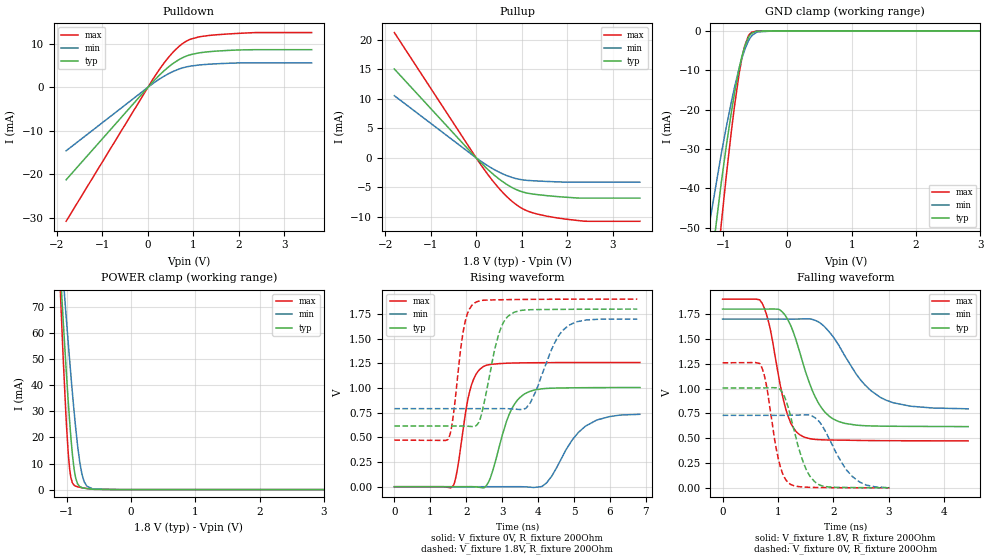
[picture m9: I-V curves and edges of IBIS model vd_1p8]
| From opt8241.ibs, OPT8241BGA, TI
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|   vd_1p8 Model
[Model]   vd_1p8
Model_type   I/O
Polarity   Non-Inverting
Enable   Active-Low
Vinl = 0.54
Vinh = 1.26
Vmeas = 0.9
Vref = 0
Cref = 2pF
Rref = 300
|   typ   min   max
|   (nom PVT)   (fast PVT)   (slow PVT)
C_comp   2.314e-12   2.106e-12   2.515e-12
[Model spec]
|subparameter
Vinl   0.54   0.51   0.57
Vinh   1.26   1.19   1.33
| Where nom  PVT is Nominal Process, 1.8V, 27C
|   Fast PVT is Strong Process,  1.9V, -40C
|   Slow PVT is Weak Process,   1.7V, 125C
[Voltage Range]   1.8   1.7   1.9
|Junction Temperature
[Temperature Range]   27   125   -40
[Pullup Reference]   1.8   1.7   1.9
[Pulldown Reference]   0   0   0
[Power Clamp Reference]   1.8   1.7   1.9
[GND Clamp Reference]   0   0   0
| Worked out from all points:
|   slope of the pulldown table from 0 to 0.27 V, typ, clamps not added: 90.7 ohm
|   slope of the pullup table from 0 to 0.27 V, typ, clamps not added: 131 ohm
|   GND clamp passes 1 mA (typ) near -0.58 V on its own axis
|   POWER clamp passes 1 mA (typ) near -0.78 V on its own axis
|   falling waveform, V_fixture 1.8V, R_fixture 200Ohm: 20-80 % time 451ps typ, 685ps min, 306ps max; typ from 1.8 V to 0.617 V
|   rising waveform, V_fixture 0V, R_fixture 200Ohm: 20-80 % time 523ps typ, 792ps min, 341ps max; typ from 0 V to 1 V
|   rising waveform, V_fixture 1.8V, R_fixture 200Ohm: 20-80 % time 422ps typ, 606ps min, 286ps max; typ from 0.614 V to 1.8 V
|   falling waveform, V_fixture 0V, R_fixture 200Ohm: 20-80 % time 309ps typ, 448ps min, 225ps max; typ from 1.01 V to 0.002 V
[Pulldown]
|   Voltage   I(typ)   I(min)   I(max)
-1.8V     -21.3mA    -14.64mA   -30.86mA
138.6mV   1.594mA    1.077mA    2.336mA
321.6mV   3.491mA    2.343mA    5.13mA
467.8mV   4.81mA     3.206mA    7.084mA
579.6mV   5.682mA    3.765mA    8.38mA
736.5mV   6.676mA    4.382mA    9.863mA
943.6mV   7.528mA    4.886mA    11.09mA
1.147V    7.957mA    5.151mA    11.65mA
1.464V    8.296mA    5.386mA    12.05mA
2.379V    8.654mA    5.601mA    12.6mA
3.6V      8.654mA    5.601mA    12.6mA
[GND Clamp]
|   Voltage   I(typ)   I(min)   I(max)
-1.8V     -229.4mA   -136.4mA   -324.1mA
-1.234V   -65.48mA   -50.91mA   -83.76mA
-1.03V    -38.61mA   -31.28mA   -49.11mA
-872.8mV  -20.69mA   -18.03mA   -25.55mA
-756.2mV  -9.942mA   -9.797mA   -11.38mA
-710.3mV  -6.6mA     -7.091mA   -7.076mA
-663.8mV  -3.897mA   -4.757mA   -3.745mA
-604.9mV  -1.604mA   -2.501mA   -1.231mA
-552.6mV  -571.6uA   -1.205mA   -335.5uA
-474mV    -83.6uA    -300.2uA   -29.97uA
-180mV    0A         -257.9nA   0A
3.6V      0A         0A         0A
[Pullup]
|   Voltage   I(typ)   I(min)   I(max)
-1.8V     15.04mA    10.52mA    21.2mA
127.8mV   -1.011mA   -694.5uA   -1.444mA
340.3mV   -2.541mA   -1.729mA   -3.653mA
510.4mV   -3.613mA   -2.435mA   -5.227mA
682.2mV   -4.533mA   -3.019mA   -6.61mA
863.8mV   -5.298mA   -3.474mA   -7.809mA
1.049V    -5.821mA   -3.744mA   -8.708mA
1.246V    -6.112mA   -3.865mA   -9.296mA
1.563V    -6.39mA    -3.983mA   -9.866mA
1.976V    -6.655mA   -4.105mA   -10.36mA
2.389V    -6.795mA   -4.106mA   -10.71mA
3.6V      -6.795mA   -4.106mA   -10.72mA
[POWER Clamp]
|   Voltage   I(typ)   I(min)   I(max)
-1.8V     411mA      341.7mA    540.9mA
-1.105V   86.59mA    98.07mA    80.06mA
-1.067V   70.27mA    85.51mA    57.79mA
-1.012V   47.3mA     67.39mA    28.39mA
-975.5mV  33.65mA    56.1mA     13.87mA
-935.5mV  20.27mA    44.06mA    4.743mA
-880.3mV  7.155mA    28.72mA    1.602mA
-831mV    2.23mA     16.99mA    1.098mA
-763mV    752.5uA    5.919mA    741.6uA
-688.2mV  401uA      1.367mA    429.5uA
-599.2mV  175.8uA    309.4uA    159uA
3.6V      0A         0A         0A
[Ramp]
R_load = 200
|   typ   min   max
dV/dt_r   0.603657/5.22202e-10   0.438286/7.7537e-10   0.755458/3.39341e-10
dV/dt_f   0.711295/4.52207e-10   0.545564/6.91155e-10   0.856494/3.0524e-10
[Falling Waveform]
V_fixture = 1.8V
V_fixture_min = 1.7V
V_fixture_max = 1.9V
R_fixture = 200Ohm
|   Time   V(typ)   V(min)   V(max)
0s        1.8V       1.7V       1.9V
712ps     1.8V       1.7V       1.86V
858ps     1.8V       1.7V       1.605V
1.152ns   1.718V     1.7V       771.6mV
1.396ns   1.359V     1.7V       533.7mV
1.722ns   861.5mV    1.674V     486.3mV
2.092ns   668.7mV    1.44V      481.3mV
2.51ns    627.9mV    1.074V     477.6mV
2.95ns    621.2mV    883mV      475.5mV
4.43ns    617.3mV    796.2mV    473.8mV
[Rising Waveform]
V_fixture = 0V
V_fixture_min = 0V
V_fixture_max = 0V
R_fixture = 200Ohm
|   Time   V(typ)   V(min)   V(max)
0s        1.016nV    46.74nV    574.5pV
1.654ns   -3.413uV   -7.315uV   20.4mV
2.098ns   427.4uV    -11.8uV    968.1mV
2.492ns   -11.55mV   -16.66uV   1.22V
2.672ns   89.04mV    -19.16uV   1.238V
3.194ns   731.1mV    148.2uV    1.252V
3.624ns   940.3mV    -780.4uV   1.255V
4.216ns   995.1mV    32.27mV    1.257V
5.316ns   1.003V     612.7mV    1.258V
6.834ns   1.005V     733.8mV    1.259V
[Rising Waveform]
V_fixture = 1.8V
V_fixture_min = 1.7V
V_fixture_max = 1.9V
R_fixture = 200Ohm
|   Time   V(typ)   V(min)   V(max)
0s        614.5mV    790.7mV    472.3mV
1.494ns   614.5mV    790.7mV    478.9mV
1.614ns   614.5mV    790.7mV    650.7mV
1.95ns    614.2mV    790.7mV    1.638V
2.242ns   610.9mV    790.7mV    1.863V
2.91ns    1.551V     791mV      1.893V
3.158ns   1.725V     790.4mV    1.895V
3.786ns   1.793V     851.6mV    1.898V
4.84ns    1.797V     1.633V     1.899V
6.76ns    1.799V     1.699V     1.9V
[Falling Waveform]
V_fixture = 0V
V_fixture_min = 0V
V_fixture_max = 0V
R_fixture = 200Ohm
|   Time   V(typ)   V(min)   V(max)
0s        1.006V     730.5mV    1.259V
698ps     1.006V     730.4mV    1.224V
794ps     1.007V     730.3mV    1.024V
1.01ns    1.005V     730.2mV    283.9mV
1.108ns   928.3mV    730.5mV    113mV
1.198ns   783.1mV    731.1mV    46.64mV
1.468ns   239.7mV    734.7mV    8.638mV
1.706ns   42.82mV    689.2mV    4.175mV
2.342ns   3.746mV    114.3mV    1.568mV
3.01ns    1.504mV    3.202mV    622uV
